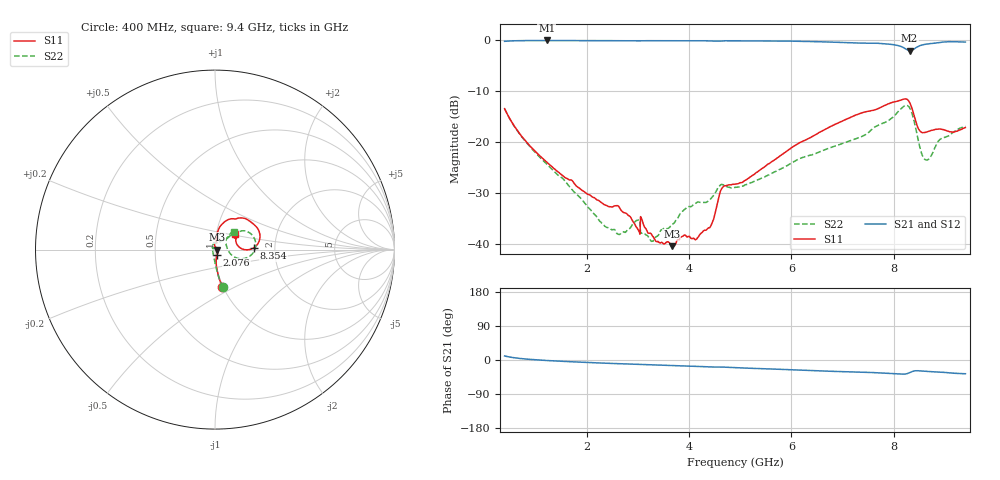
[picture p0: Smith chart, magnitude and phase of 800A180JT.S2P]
!  American Technical Ceramics  Date:  12/17/08
!  One Norden Lane
!  Huntington Station,  NY.  11746-2102
!  Tel:  (631) 622-4700  Fax:  (631) 622-4748
!  Part Number  800A180JT
!  Description: Broardband capacitor  Mounting Orientation: Vertical
!  Application:
# GHZ S DB R 50
! Freq  |S11|  S11 Ph  |S21|  S21 Ph  |S12|  S12 Ph  |S22|  S22 Ph
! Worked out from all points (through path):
!   801 points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, 400 MHz to 9.4 GHz, reference 50 ohm
!   highest |S21| = -0.06 dB at 1.221 GHz (marker M1); lowest = -2.0 dB at 8.309 GHz (marker M2)
!   group delay of S21, straight-line fit = 12.7 ps
!   lowest |S11| = -40.3 dB at 3.663 GHz (marker M3), VSWR 1.02, Z = 51 + j0.047 ohm
!   |S11| at or under -10 dB: start of sweep to end of sweep
!   |S22| runs from -39.4 to -12.8 dB; largest |S21 - S12| = 0.0054
!   S11 on the Smith chart (normalised r, x): 400 MHz: 0.99, -0.43; 2.076 GHz: 1.02, -0.06; 8.354 GHz: 1.55, +0.03; 9.4 GHz: 1.23, +0.21
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0.4  -13.42 -78.8  -0.23 10.7  -0.21 10.7  -13.42 -78.5
1.221  -23.90 -84.3  -0.06 -1.3  -0.04 -1.4  -24.29 -92.3
1.908  -29.39 -72.9  -0.07 -5.8  -0.05 -5.9  -31.19 -110.7
2.076  -30.38 -66.8  -0.08 -6.8  -0.06 -6.8  -33.18 -118.9
2.616  -32.44 -45.5  -0.12 -9.6  -0.10 -9.7  -37.97 178.7
2.999  -36.99 -30.2  -0.14 -11.4  -0.12 -11.5  -35.27 129.7
3.1  -35.71 -57.5  -0.13 -11.7  -0.11 -11.8  -37.76 147.2
3.258  -37.88 -40.6  -0.10 -12.5  -0.09 -12.6  -39.28 142.6
3.404  -39.51 -25.0  -0.09 -13.3  -0.07 -13.4  -38.18 152.7
3.663  -40.34 2.8  -0.10 -14.6  -0.09 -14.7  -36.14 146.0
3.955  -38.44 26.4  -0.12 -16.0  -0.11 -16.1  -32.80 133.8
4.383  -36.75 74.0  -0.14 -18.1  -0.13 -18.2  -31.49 112.2
4.641  -29.06 89.0  -0.17 -18.6  -0.16 -18.8  -28.25 92.8
4.9  -28.18 74.7  -0.11 -20.2  -0.10 -20.3  -28.83 75.4
6.408  -18.88 80.2  -0.28 -27.9  -0.28 -28.1  -22.44 44.9
7.904  -12.44 46.8  -0.78 -35.4  -0.79 -35.6  -15.71 37.1
8.309  -12.18 9.3  -2.05 -33.6  -2.06 -33.8  -13.21 -2.3
8.354  -13.27 2.8  -1.98 -30.9  -2.00 -31.1  -14.25 -11.6
8.5  -17.63 8.2  -1.13 -28.5  -1.15 -28.7  -20.52 -17.1
8.635  -18.02 22.9  -0.78 -29.9  -0.79 -30.2  -23.45 14.4
8.916  -17.41 27.8  -0.44 -32.0  -0.46 -32.2  -19.35 43.2
9.4  -17.11 37.2  -0.37 -36.2  -0.40 -36.5  -16.88 43.9
